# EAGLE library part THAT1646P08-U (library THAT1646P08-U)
IC, LINE DRIVER, BALANCED, 1CH, 8DIP Source: Datasheet
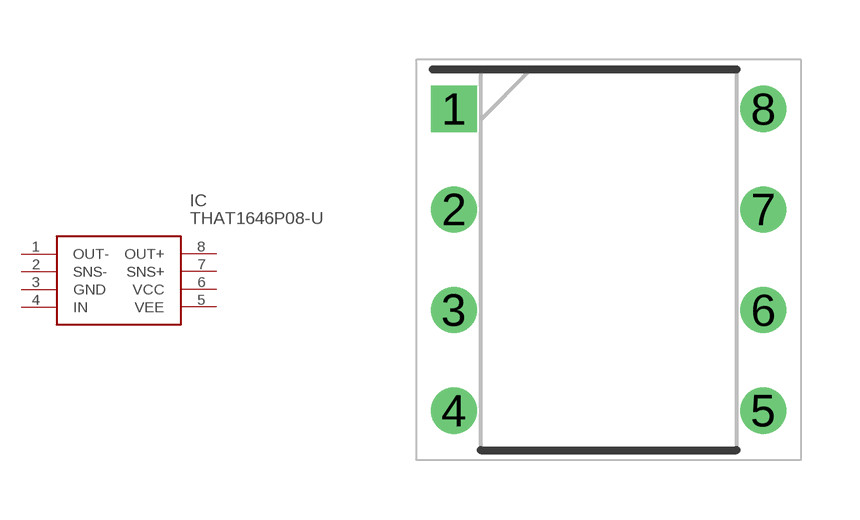
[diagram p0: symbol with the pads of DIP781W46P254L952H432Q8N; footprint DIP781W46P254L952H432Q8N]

Designator prefix IC

## THAT1646P08-U (Description: IC, LINE DRIVER, BALANCED, 1CH, 8DIP; Height: 4.32mm; Manufacturer_Name: THAT CORPORATION; Manufacturer_Part_Number: THAT1646P08-U)  [DIP781W46P254L952H432Q8N]
1  OUT-
2  SNS-
3  GND
4  IN
5  VEE
6  VCC
7  SNS+
8  OUT+

## Footprint DIP781W46P254L952H432Q8N (pad centres in mm)
8 DIP_1
drill 0.66 pad 1.06 square: 1 -3.905,3.81
drill 0.66 pad 1.06: 2 -3.905,1.27; 3 -3.905,-1.27; 4 -3.905,-3.81; 5 3.905,-3.81; 6 3.905,-1.27; 7 3.905,1.27; 8 3.905,3.81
